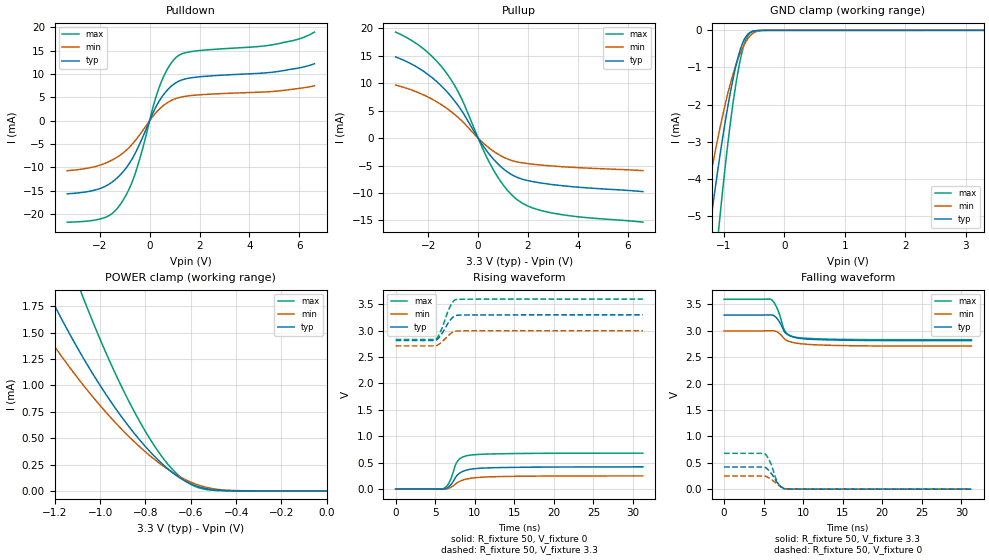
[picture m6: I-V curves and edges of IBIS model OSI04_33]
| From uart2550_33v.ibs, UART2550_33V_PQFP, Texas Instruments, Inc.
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[Model]   OSI04_33
Model_type  3-state
Enable   Active-Low
Vref =   1.65
Rref =   50
Cref =   15p
Vmeas =   1.65
| variable   typ   min   max
C_comp   0.94pF   0.62pF   1.17pF
| C_pullup   1.17pF   0.61pF   1.55pF
| C_pulldown   1.11pF   0.74pF   1.38pF
| C_tri-state   0.94pF   0.62pF   1.17pF
[Temperature Range]   40   125   -40
| Ambient temperature   25   110   -40
[Voltage range]   3.3   3   3.6
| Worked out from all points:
|   slope of the pulldown table from 0 to 0.495 V, typ, clamps not added: 96.6 ohm
|   slope of the pullup table from 0 to 0.495 V, typ, clamps not added: 154 ohm
|   GND clamp passes 1 mA (typ) near -0.81 V on its own axis
|   POWER clamp passes 1 mA (typ) near -1.00 V on its own axis
|   rising waveform, R_fixture 50, V_fixture 0: 20-80 % time 1.52ns typ, 2.15ns min, 1.11ns max; typ from 0.001 V to 0.42 V
|   falling waveform, R_fixture 50, V_fixture 3.3: 20-80 % time 1.4ns typ, 2.05ns min, 1.09ns max; typ from 3.3 V to 2.81 V
|   rising waveform, R_fixture 50, V_fixture 3.3: 20-80 % time 1.21ns typ, 1.23ns min, 1.17ns max; typ from 2.81 V to 3.3 V
|   falling waveform, R_fixture 50, V_fixture 0: 20-80 % time 1.16ns typ, 1.31ns min, 1.01ns max; typ from 0.42 V to 0.001 V
[GND Clamp]
| OSI04_33
|   Voltage   I(typ)   I(min)   I(max)
-3.3V     -39.47mA   -29.89mA   -53.49mA
-1.37V    -7.137mA   -5.341mA   -10.51mA
-1.335V   -6.669mA   -5.001mA   -9.836mA
-1.215V   -5.131mA   -3.893mA   -7.61mA
-1.075V   -3.493mA   -2.721mA   -5.198mA
-915mV    -1.881mA   -1.583mA   -2.801mA
-795mV    -922.5uA   -909.5uA   -1.396mA
-675mV    -290.6uA   -423uA     -443uA
-620mV    -137.4uA   -265uA     -198.8uA
-555mV    -46.8uA    -131.2uA   -59.04uA
-340mV    -475.9nA   -2.499uA   -272.3nA
3.3V      184.3pA    357.4nA    130.9pA
[POWER Clamp]
| OSI04_33
|   Voltage   I(typ)   I(min)   I(max)
-3.3V     16.63mA    12.21mA    22.69mA
-1.345V   2.395mA    1.835mA    3.527mA
-1.215V   1.814mA    1.411mA    2.662mA
-1.075V   1.261mA    1.004mA    1.832mA
-955mV    852.3uA    698.9uA    1.215mA
-840mV    520.4uA    447.1uA    713.8uA
-730mV    264.4uA    248.5uA    332.3uA
-640mV    112.5uA    124.6uA    120.1uA
-580mV    49.18uA    65.74uA    41.5uA
-510mV    13.32uA    23.88uA    7.159uA
-405mV    1.164uA    3.277uA    270.7nA
-47.99fV  184.3pA    793.1pA    148.1pA
[Pulldown]
| OSI04_33
|   Voltage   I(typ)   I(min)   I(max)
-3.3V     -15.64mA   -10.69mA   -21.7mA
-1.815V   -14.14mA   -9.184mA   -20.76mA
-1.12V    -11.27mA   -7.131mA   -17.5mA
-810mV    -9.133mA   -5.679mA   -14.51mA
-555mV    -6.742mA   -4.118mA   -10.95mA
165mV     1.997mA    1.163mA    3.441mA
415mV     4.449mA    2.606mA    7.558mA
755mV     6.804mA    3.992mA    11.42mA
1.11V     8.296mA    4.845mA    13.76mA
1.825V    9.299mA    5.469mA    14.91mA
4.975V    10.41mA    6.281mA    16.3mA
6.6V      12.19mA    7.474mA    18.96mA
[Pullup]
| OSI04_33
|   Voltage   I(typ)   I(min)   I(max)
-3.3V     14.79mA    9.667mA    19.31mA
-2.165V   12.12mA    7.837mA    16.19mA
-1.69V    10.44mA    6.71mA     14.19mA
-1.26V    8.519mA    5.444mA    11.82mA
-680mV    5.156mA    3.277mA    7.387mA
155mV     -1.076mA   -669.4uA   -1.602mA
580mV     -3.641mA   -2.262mA   -5.495mA
1.075V    -5.815mA   -3.586mA   -8.927mA
1.58V     -7.171mA   -4.346mA   -11.26mA
2.175V    -7.899mA   -4.735mA   -12.69mA
3.09V     -8.523mA   -5.117mA   -13.74mA
6.6V      -9.745mA   -5.926mA   -15.31mA
[Ramp]
| OSI04_33
| variable   typ   min   max
dV/dt_r   0.25/1.51E-09   0.15/2.17E-09   0.39/1.09E-09
dV/dt_f   0.29/1.39E-09   0.17/2.06E-09   0.43/1.03E-09
R_load = 50
[Rising Waveform]
| OSI04_33
R_fixture =   50
C_fixture =   0
L_fixture =   0
V_fixture =   0
V_fixture_min = 0
V_fixture_max = 0
|   Time   V(typ)   V(min)   V(max)
0s        755.2uV    577.9uV    986.2uV
6.08ns    771.2uV    -1.718mV   10.63mV
6.505ns   23.76mV    6.777mV    64.71mV
6.835ns   60.98mV    23.45mV    144.4mV
7.555ns   214.7mV    94.97mV    453.4mV
7.83ns    267.6mV    124.1mV    528.4mV
8.435ns   331.2mV    165.9mV    602.4mV
9.325ns   371.7mV    199.5mV    639.9mV
14.43ns   409.6mV    239.6mV    671.2mV
31.25ns   419.7mV    249.2mV    679.5mV
[Falling Waveform]
| OSI04_33
R_fixture =   50
C_fixture =   0
L_fixture =   0
V_fixture =   3.3
V_fixture_min = 3
V_fixture_max = 3.6
|   Time   V(typ)   V(min)   V(max)
0s        3.299V     2.999V     3.599V
5.975ns   3.302V     3.003V     3.593V
6.325ns   3.285V     3V         3.533V
6.745ns   3.224V     2.977V     3.412V
7.51ns    3.017V     2.867V     3.051V
7.7ns     2.969V     2.839V     2.993V
8.26ns    2.91V      2.798V     2.918V
9.23ns    2.866V     2.766V     2.875V
15.24ns   2.823V     2.721V     2.838V
31.25ns   2.814V     2.712V     2.832V
[Rising Waveform]
| OSI04_33
R_fixture =   50
C_fixture =   0
L_fixture =   0
V_fixture =   3.3
V_fixture_min = 3
V_fixture_max = 3.6
|   Time   V(typ)   V(min)   V(max)
0s        2.814V     2.712V     2.832V
5.085ns   2.817V     2.713V     2.837V
5.36ns    2.849V     2.732V     2.89V
5.715ns   2.915V     2.772V     2.997V
6ns       2.98V      2.809V     3.104V
6.555ns   3.125V     2.892V     3.344V
6.9ns     3.2V       2.939V     3.46V
7.28ns    3.26V      2.976V     3.555V
7.625ns   3.289V     2.991V     3.589V
31.25ns   3.299V     2.999V     3.599V
[Falling Waveform]
| OSI04_33
R_fixture =   50
C_fixture =   0
L_fixture =   0
V_fixture =   0
V_fixture_min = 0
V_fixture_max = 0
|   Time   V(typ)   V(min)   V(max)
0s        420.2mV    249.6mV    679.7mV
5.115ns   417.8mV    248.8mV    674.8mV
5.43ns    387.6mV    233.2mV    622.3mV
5.825ns   325.3mV    199.6mV    513.9mV
6.475ns   179.5mV    125.3mV    228.2mV
6.795ns   107.6mV    85.24mV    120.1mV
7.195ns   46.18mV    45.18mV    39.9mV
7.6ns     12.22mV    18.16mV    8.148mV
9.325ns   2.257mV    2.045mV    2.604mV
31.25ns   779.7uV    593.2uV    996.6uV
